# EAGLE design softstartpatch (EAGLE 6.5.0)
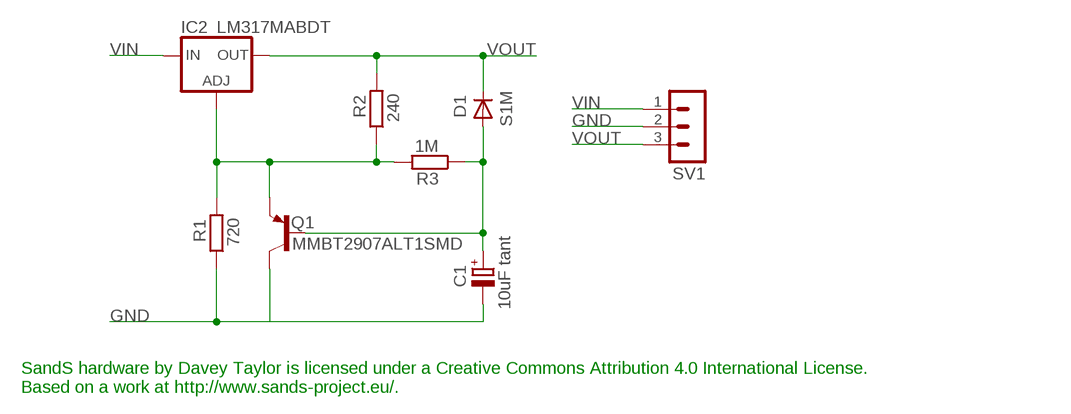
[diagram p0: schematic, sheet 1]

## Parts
C1  10uF tant  CPOL-EUSMCB  [SMC_B]
D1  S1M  DIODE-SMB  [SMB]
IC2  LM317MABDT  [DPACK]
Q1  MMBT2907ALT1SMD  [SOT23-BEC]
R1  720  R-EU_R0603  [R0603]
R2  240  R-EU_R0603  [R0603]
R3  1M  R-EU_R0603  [R0603]
SV1  MA03-1  [MA03-1]

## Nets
GND: C1.- Q1.C R1.1 SV1.2
N$2: IC2.1(ADJ) Q1.E R1.2 R2.1 R3.2
N$5: C1.+ D1.A Q1.B R3.1
VIN: IC2.3(IN) SV1.1
VOUT: D1.C IC2.4(OUT) R2.2 SV1.3

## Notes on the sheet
- SandS hardware by Davey Taylor is licensed under a Creative Commons Attribution 4.0 International License.
  Based on a work at http://www.sands-project.eu/.

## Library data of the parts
C1 = rcl:CPOL-EU: POLARIZED CAPACITOR, European symbol
D1 = diode:DIODE-: DIODE
IC2 = v-reg:LM317?*: 500 mA Adjustable Output Positive Voltage Regulator Source: http://www.onsemi.co.jp .. LM317M-D.PDF
Q1 = transistor-pnp:MMBT2907*: PNP Transistror
R1-R3 = rcl:R-EU_: RESISTOR, European symbol
SV1 = con-lstb:MA03-1: PIN HEADER; OC_FARNELL: unknown; OC_NEWARK: unknown

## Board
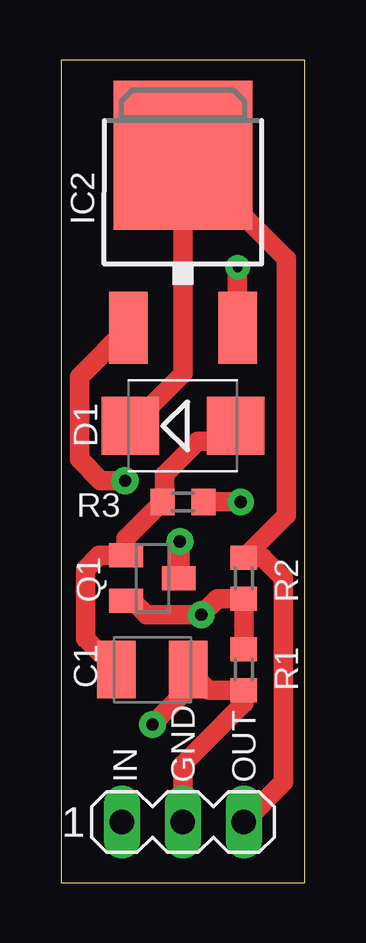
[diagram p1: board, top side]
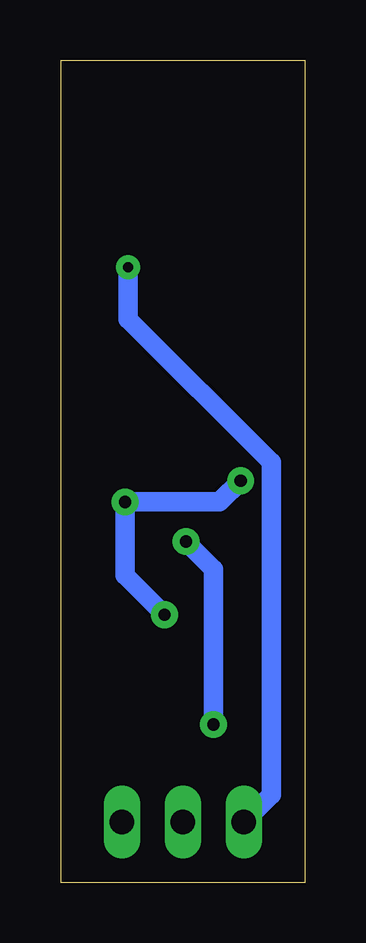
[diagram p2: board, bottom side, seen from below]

Size 10.16 x 34.29 mm. Coordinates in mm from the lower left corner, seen from the top.
Outline: 0,0 10.16,0 10.16,34.29 0,34.29 0,0
Copper layers (1*16): Top 0.035mm / dielectric 1.5mm / Bottom 0.035mm
Design rules "default": minimum track width 10mil, minimum drill 24mil, track to track 8mil, track to pad 8mil, pad to pad 8mil, via to via 8mil, smd to smd 8mil, copper to edge 40mil, drill to drill 8mil, minimum pad ring 10mil, minimum via ring 8mil, stop-mask expansion 4mil, vias tented up to drill 0mil, thermal gap 10mil

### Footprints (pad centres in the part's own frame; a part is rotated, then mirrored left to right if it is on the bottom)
SMC_B = smd 1.6 x 2.4: + -1.5,0; - 1.5,0
SMB = smd 2.4 x 2.4: A 2.2,0; C -2.2,0
DPACK = smd 1.6 x 3: 1 -2.28,-4.8; 3 2.28,-4.8 | smd 5.8 x 6.2: 4 0,2.38
SOT23-BEC = smd 1 x 1.4: B -0.95,-1.1; C 0,1.1; E 0.95,-1.1
R0603 = smd 1 x 1.1: 1 -0.85,0; 2 0.85,0
MA03-1 = drill 1.016 long: 1 -2.54,0; 2 0,0; 3 2.54,0

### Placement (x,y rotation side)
C1  3.81,8.89 0 top
D1  5.08,19.05 0 top
IC2  5.08,27.94 0 top
Q1  3.81,12.7 270 top
R1  7.62,8.89 90 top
R2  7.62,12.7 90 top
R3  5.08,15.88 0 top
SV1  5.08,2.54 0 top

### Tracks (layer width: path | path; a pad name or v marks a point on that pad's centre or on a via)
GND  (via drill 0.51 pad 1.12)
  Top 0.813: Q1.C 4.95,12.74 v4.95,14.22 | v3.81,6.6 5.33,8.13 C1.- 6.16,8.04 R1.1 7.62,7.49 5.08,4.95 SV1.2
  Bottom 0.813: v4.95,14.22 3.81,13.08 v3.81,6.6
N$2  (via drill 0.51 pad 1.12)
  Top 0.813: v2.67,16.76 1.65,16.76 0.76,17.65 0.76,21.1 IC2.1 | R1.2 R2.1 6.52,11.85 v5.84,11.18 3.56,11.18 2.98,11.75 Q1.E | R3.2 v7.49,15.88
  Bottom 0.813: v2.67,16.76 3.56,15.88 v7.49,15.88 7.49,12.83 v5.84,11.18
N$5
  Top 0.813: C1.+ 1.02,10.18 1.02,13.08 1.58,13.65 Q1.B 2.71,14.36 R3.1 4.32,15.79 4.32,17.02 5.71,18.41 6.64,18.41 D1.A
VIN  (via drill 0.41 pad 1.02)
  Top 0.813: IC2.3 v7.36,25.65 v7.37,25.65
  Bottom 0.813: v7.37,25.65 7.37,23.5 1.4,17.53 1.4,3.68 SV1.1
VOUT
  Top 0.813: D1.C 2.54,18.71 2.54,18.67 5.08,21.21 IC2.4 9.4,26 9.4,15.33 R2.2 8.42,13.55 9.27,12.7 9.27,4.19 SV1.3

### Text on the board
tNames: IN | GND | OUT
